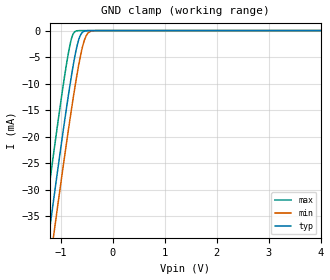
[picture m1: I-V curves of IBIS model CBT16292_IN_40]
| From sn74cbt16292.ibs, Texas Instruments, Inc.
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[Model]   CBT16292_IN_40
Model_type  Input
Vinl = 0.8
Vinh = 2.0
| variable   typ   min   max
C_comp   1.43pF   1.10pF   1.75pF
[Temperature Range]   40   100   -40
| Ambient temperature   25   85   -40
[Voltage range]   4   4   4
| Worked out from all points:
|   GND clamp passes 1 mA (typ) near -0.63 V on its own axis
[GND Clamp]
| CBT16292_IN_40
|   Voltage   I(typ)   I(min)   I(max)
-4V       -250mA     -256.3mA   -242mA
-1.365V   -48.74mA   -55.5mA    -40.02mA
-1.31V    -44.67mA   -51.45mA   -35.94mA
-1.21V    -37.33mA   -44.12mA   -28.58mA
-1.125V   -31.16mA   -37.95mA   -22.41mA
-850mV    -12.12mA   -18.65mA   -4.156mA
-780mV    -7.787mA   -14.05mA   -1.143mA
-710mV    -4.013mA   -9.713mA   -111.7uA
-630mV    -1.091mA   -5.305mA   -4.37uA
-555mV    -159.3uA   -2.168mA   -194.1nA
-405mV    -1.677uA   -91.86uA   -391.1pA
4V        28.91pA    2.706nA    22.55pA
